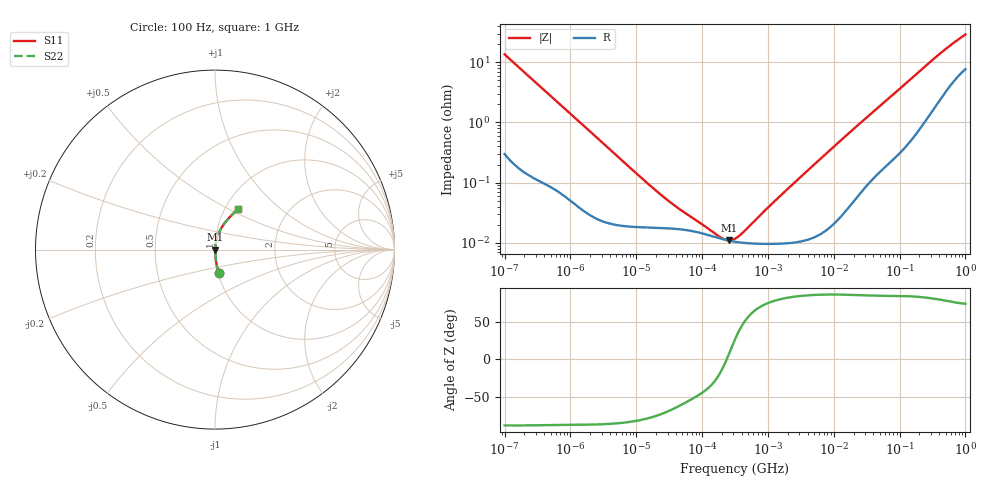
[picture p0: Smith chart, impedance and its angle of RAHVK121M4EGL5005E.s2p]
! RAHVK121M4EGL5005E  S-PARAMETER MODEL  (AEC-Q200 qualified)
! Model Generated by ELNA Corporation (http://www.ty-top.com)
! Version 1.0
! ELNA Control No. 201214
! Copyright (c) 2020 ELNA CO.,LTD. All Rights Reserved.
! Products Name : CONDUCTIVE POLYMER HYBRID ALUMINUM ELECTROLYTIC CAPACITORS
! Characteristics :
!  Capacitance  :  120uF  ,  Rated voltage  :  63V
!  Operating Temp. Range  :  -55 to +125 degC  ,  Endurance  :  4000hr at 125 degC
!  Dimension D  :  12.5mm  ,  Dimension L  :  13.5mm
! Frequency Range : 100Hz - 1GHz
! External Node Assignments :
!  1  o---| |---o  2
# MHz S RI R 50
!Freq[MHz].  S11 Real  S11 Imag  S21 Real  S21 Imag  S12 Real  S12 Imag  S22 Real  S22 Imag
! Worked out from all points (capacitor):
!   401 points, 100 Hz to 1 GHz, reference 50 ohm
!   read as one part in series: C = 118 uF near 108 Hz
!   lowest |Z| = 11 mohm at 258.5 kHz (marker M1)
!   series resonance near 236.8 kHz, so ESL is about 3.8 nH
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0.0001  0.0207 -0.1319  0.9793 0.1319  0.9793 0.1319  0.0207 -0.1319
0.000113  0.0166 -0.1175  0.9834 0.1175  0.9834 0.1175  0.0166 -0.1175
0.000183  0.00699 -0.0734  0.993 0.0734  0.993 0.0734  0.00699 -0.0734
0.000309  0.00304 -0.0438  0.997 0.0438  0.997 0.0438  0.00304 -0.0438
0.001488  0.000446 -0.00941  0.9996 0.00941  0.9996 0.00941  0.000446 -0.00941
0.010292  0.000185 -0.00138  0.9998 0.00138  0.9998 0.00138  0.000185 -0.00138
0.022131  0.000177 -0.000645  0.9998 0.000645  0.9998 0.000645  0.000177 -0.000645
0.043904  0.000169 -0.000332  0.9998 0.000332  0.9998 0.000332  0.000169 -0.000332
0.179887  0.00012 -4.64e-05  0.9999 4.64e-05  0.9999 4.64e-05  0.00012 -4.64e-05
0.220039  0.000113 -1.26e-05  0.9999 1.26e-05  0.9999 1.26e-05  0.000113 -1.26e-05
0.258523  0.000109 1.55e-05  0.9999 -1.55e-05  0.9999 -1.55e-05  0.000109 1.55e-05
0.316228  0.000104 5.27e-05  0.9999 -5.27e-05  0.9999 -5.27e-05  0.000104 5.27e-05
0.419276  0.0001 0.00011  0.9999 -0.00011  0.9999 -0.00011  0.0001 0.00011
1.195364  9.63e-05 0.000454  0.9999 -0.000454  0.9999 -0.000454  9.63e-05 0.000454
4.704354  0.000123 0.00186  0.9999 -0.00186  0.9999 -0.00186  0.000123 0.00186
18.51399  0.000489 0.00721  0.9995 -0.00721  0.9995 -0.00721  0.000489 0.00721
69.9842  0.00275 0.0254  0.9972 -0.0254  0.9972 -0.0254  0.00275 0.0254
169.8244  0.00947 0.0591  0.9905 -0.0591  0.9905 -0.0591  0.00947 0.0591
380.1894  0.0357 0.1207  0.9643 -0.1207  0.9643 -0.1207  0.0357 0.1207
641.9482  0.0774 0.1758  0.9226 -0.1758  0.9226 -0.1758  0.0774 0.1758
922.5714  0.1192 0.2163  0.8808 -0.2163  0.8808 -0.2163  0.1192 0.2163
1000  0.1297 0.2255  0.8703 -0.2255  0.8703 -0.2255  0.1297 0.2255
